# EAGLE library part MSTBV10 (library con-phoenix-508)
PHOENIX
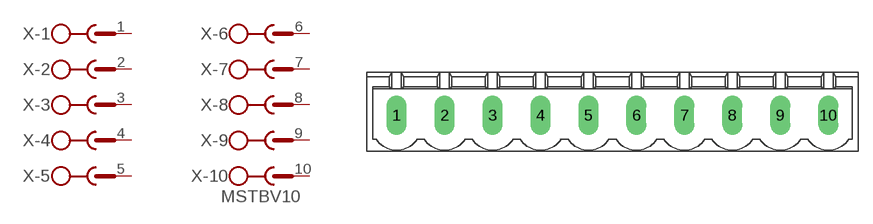
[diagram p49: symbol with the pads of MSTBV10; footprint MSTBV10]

Designator prefix X; gates -1=SK -2=SK -3=SK -4=SK -5=SK -6=SK -7=SK -8=SK -9=SK -10=SKV

## MSTBV10 (MPN: MSTBV 2,5/10-GF-5.08; OC_FARNELL: 1792798; OC_NEWARK: 69R9844)  [MSTBV10]
1  -1:1  pas
2  -2:1  pas
3  -3:1  pas
4  -4:1  pas
5  -5:1  pas
6  -6:1  pas
7  -7:1  pas
8  -8:1  pas
9  -9:1  pas
10  -10:1  pas

## Footprint MSTBV10 (pad centres in mm)
PHOENIX
drill 1.397 long: 1 -22.86,0; 2 -17.78,0; 3 -12.7,0; 4 -7.62,0; 5 -2.54,0; 6 2.54,0; 7 7.62,0; 8 12.7,0; 9 17.78,0; 10 22.86,0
